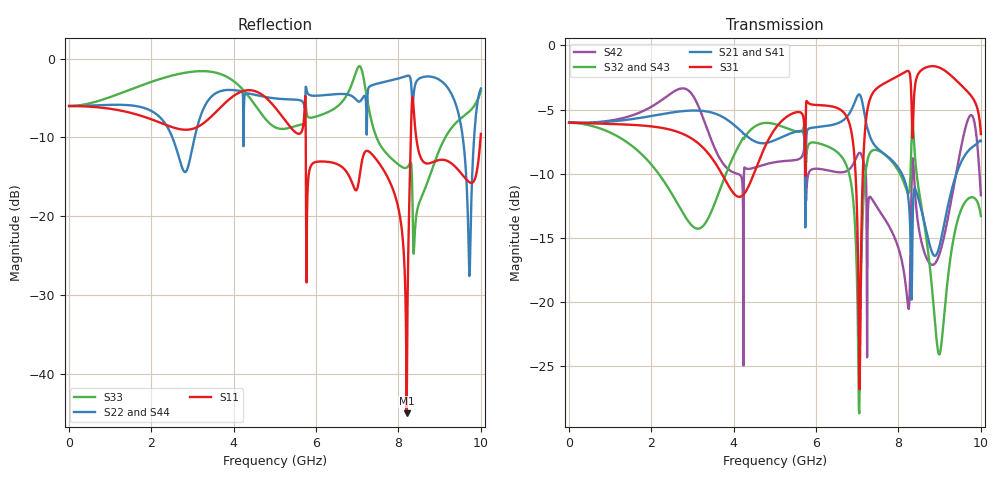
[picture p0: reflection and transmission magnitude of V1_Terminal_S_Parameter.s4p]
! Touchstone file exported from HFSS 2022.1.0
!  File:  C:/Users/Tatjana/Downloads/Sorted/ReI_project_FLPP_PPM/_TS/_microstrip/HFSS/V01/V1.aedt
!  Generated:  12:03:04 p%xE7cp.  j%xFBl. 24, 2024
!  Design:  HFSSDesign1
!  Project:  V1
!  Setup:  Setup1
!  Solution:  Sweep
! Variables:
!  $Dx = 2mm
!  $Dy = 2mm
!  $Dz = 5mm
!  $Dz_neg = 2mm
!  $L1 = 9.5mm
!  $L2 = 9.2mm
!  $L_cb = 10.125mm
!  $L_cb_ = 20.125mm
!  $L_delay = 0mm
!  $L_feed = 5mm
!  $L_match = 5mm
!  $L_out = 5mm
!  $L_window = 8.875mm
!  $Ls = 20.125mm
!  $R_match = 120ohm
!  $W1 = 1.15mm
!  $W2 = 1.15mm
!  $W3 = 0.9mm
!  $W4 = 0.35mm
!  $W_cb = 19.55mm
!  $W_delay = 2.9mm
!  $W_feed = 2.9mm
!  $W_match = 2.9mm
!  $W_out = 2.9mm
!  $W_window = 8.05mm
!  $Ws = 29.325mm
!  $cnc_gap = 0mm
!  $h = 1.6mm
!  $match_port_ht = 1.6mm
!  $match_port_wd = 2.9mm
!  $out_port_ht = 1.6mm
!  $out_port_wd = 2.9mm
!  $port_ht = 1.6mm
!  $port_wd = 2.9mm
# GHz S RI R 50.000000
! Terminal data exported
! Port[1] = CB_L_T1
! Port[2] = CB_L_T2
! Port[3] = CB_L_T3
! Port[4] = CB_L_T4
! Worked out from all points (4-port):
!   1000 points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, 10 MHz to 10 GHz, reference 50 ohm
!   strongest paths, dB at 10 MHz, 2.51 GHz, 5.01 GHz, 7.51 GHz, 10 GHz:
!     S31: -6.0, -6.6, -6.5, -3.3, -6.9
!     S21: -6.0, -5.2, -7.4, -8.1, -7.5
!     S41: -6.0, -5.3, -7.3, -8.1, -7.4
!     S32: -6.0, -11.6, -6.1, -8.2, -13.3
!     S43: -6.0, -11.7, -6.3, -8.2, -13.2
!     S42: -6.0, -3.7, -9.1, -12.8, -11.7
!   lowest |S11| = -45.0 dB at 8.2 GHz (marker M1), VSWR 1.01, Z = 50 - j0.559 ohm
!   |S11| at or under -10 dB: 5.751 GHz to 8.3 GHz (2.549 GHz wide, 36.3 % of centre); 8.431 GHz to 9.993 GHz (1.563 GHz wide, 17 % of centre)
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0.01  -0.4998 0.00352  0.4998 -0.00512  0.4999 -0.00488  0.4998 -0.00513
      0.4998 -0.00512  -0.4998 0.00417  0.4999 -0.00428  0.4998 -0.00637
      0.4999 -0.00488  0.4999 -0.00428  -0.4999 0.00184  0.4999 -0.00428
      0.4998 -0.00513  0.4998 -0.00637  0.4999 -0.00428  -0.4998 0.00418
3.72  0.215 0.4521  -0.2941 0.4379  0.0114 0.3141  -0.2942 0.4385
      -0.2941 0.4379  0.3426 0.5229  -0.0607 -0.2812  0.0629 -0.3451
      0.0114 0.3141  -0.0607 -0.2812  0.7785 0.14  -0.0628 -0.2782
      -0.2942 0.4385  0.0629 -0.3451  -0.0628 -0.2782  0.3449 0.523
5.34  -0.1586 -0.3426  0.3855 0.2344  -0.5275 0.0787  0.3876 0.2312
      0.3855 0.2344  -0.1914 -0.5166  -0.4417 0.166  0.0664 0.3489
      -0.5275 0.0787  -0.4417 0.166  -0.2746 0.2364  -0.4383 0.1586
      0.3876 0.2312  0.0664 0.3489  -0.4383 0.1586  -0.189 -0.5222
8.2  -0.000184 -0.00559  -0.2636 0.09  0.7285 -0.3166  -0.2596 0.0964
     -0.2636 0.09  0.7701 0.0921  0.2578 0.0873  -0.103 0.029
     0.7285 -0.3166  0.2578 0.0873  0.2017 0.0219  0.2573 0.0869
     -0.2596 0.0964  -0.103 0.029  0.2573 0.0869  0.7715 0.0679
8.35  0.2073 0.5161  -0.0454 -0.2188  0.4328 -0.185  -0.0421 -0.2335
      -0.0454 -0.2188  0.5223 -0.0369  0.4946 0.0112  -0.3314 0.1451
      0.4328 -0.185  0.4946 0.0112  -0.0721 -0.0508  0.5054 0.0033
      -0.0421 -0.2335  -0.3314 0.1451  0.5054 0.0033  0.4973 -0.0423
9.73  -0.054 -0.1544  -0.2603 0.2948  -0.5356 -0.361  -0.2712 0.2753
      -0.2603 0.2948  0.0422 -0.0125  0.1811 0.179  -0.5261 0.0677
      -0.5356 -0.361  0.1811 0.179  0.3866 -0.2575  0.1723 0.2095
      -0.2712 0.2753  -0.5261 0.0677  0.1723 0.2095  0.0143 0.015
10  -0.1588 -0.2922  -0.0473 0.4207  -0.4406 0.0975  -0.0443 0.4253
    -0.0473 0.4207  -0.6046 0.2257  0.1751 0.1263  0.242 0.0957
    -0.4406 0.0975  0.1751 0.1263  0.0407 -0.6211  0.172 0.1348
    -0.0443 0.4253  0.242 0.0957  0.172 0.1348  -0.6001 0.2323
